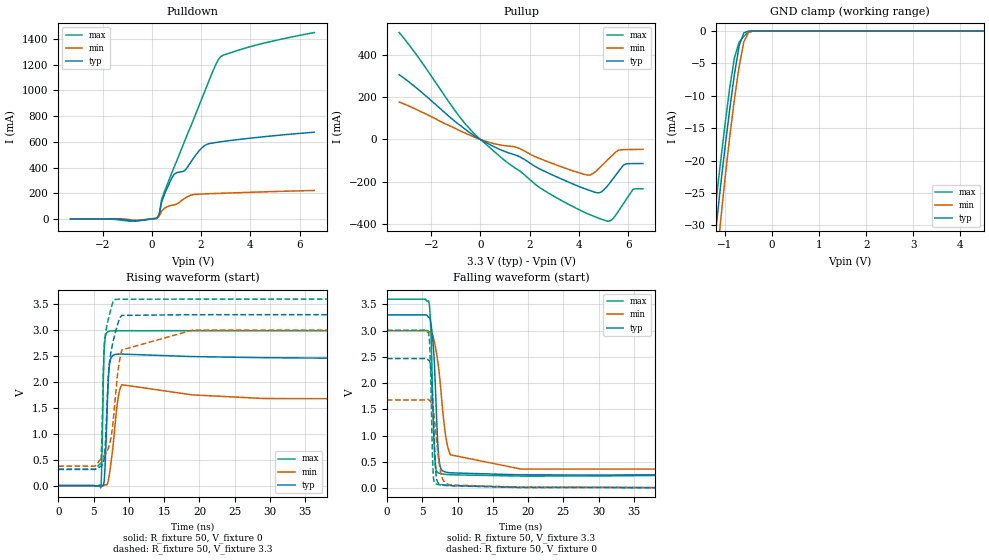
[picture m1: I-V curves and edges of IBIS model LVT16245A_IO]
|   TEXAS INSTRUMENTS INCORPORATED
|   Advanced Bus Interface Group
|   IBIS Model of SN74LVT16245A
|   3.3-V ABT 16-BIT TRANSCEIVER WITH 3-STATE OUTPUTS
[IBIS Ver]   2.1
[File Name]   sn74lvt16245a.ibs
[File Rev]   1.0
[Date]   05/30/2000
[Source]   File originated at Texas Instruments, Inc.
[Notes]   The following is an IBIS list for the LVT16245A.
|   - All test data contained in this file are derived from
|   hspice(tm) simulations.
|   -  This file may be incomplete or may not be fully compliant
   with the IBIS specification. It will be replaced with a
   version that is IBIS Revision 3.2 compliant and is complete
   and accurate. Please email all questions and comments to
   sllibis@ti.com.
[Disclaimer] Property of Texas Instruments Incorporated.  Unauthorized
   reproduction and/or distribution is strictly prohibited.
   This product is protected under copyright law.
   Created 1996, (C) Copyright 1996, Texas Instruments Inc.,
   All Rights Reserved
   UNLESS THERE IS A SIGNED, WRITTEN AGREEMENT TO THE
   CONTRARY, TEXAS INSTRUMENTS ("TI") IS PROVIDING THE IBIS
   MODELS "AS IS" AND WITHOUT ANY WARRANTY, EXPRESSED OR
   IMPLIED.  TI assumes no liability for:
   1) the accuracy of the IBIS models provided to your
   company;
   2) the proper functioning of these IBIS models in your
   design or for any resulting applications; or
   3) infringement of patents, copyrights or intellectual
   property rights resulting from your use of these IBIS
   models.
   TI provides IBIS Models as a service to our customers.
   You and your company shall not distribute, sell or give
   these models to anyone else without prior written
   permission from TI.
   TI reserves the right to make changes to our products or
   to discontinue any semiconductor product or service
   without notice, and advises our customers to obtain the
   latest version of relevant information to verify, before
   placing orders, that the information being relied on is
   current.
   Please be aware that your receipt and use of the IBIS
   information provided shall serve as acceptance of these
   terms and conditions.  If you do not accept these terms,
   you should return or destroy the IBIS models and any
   other accompanying information immediately.
[Component]   LVT16245A_DL
[manufacturer]   Texas Instruments, Inc.
[Package]
|   typ   min   max
R_pkg   0.048   0.038   0.053
L_pkg   6.046nH   5.084nH   7.968nH
C_pkg   0.813pF   0.569pF   1.157pF
[Pin] signal_name   model_name   R_pin   L_pin   C_pin
1   1DIR   NC   0.046   7.968nH   1.017pF
2   1B1   LVT16245A_IO  0.044   7.299nH   1.157pF
3   1B2   LVT16245A_IO  0.043   6.765nH   1.058pF
4   GND   GND   0.041   6.269nH   0.933pF
5   1B3   LVT16245A_IO  0.038   5.856nH   0.829pF
6   1B4   LVT16245A_IO  0.046   5.802nH   0.79pF
7   VCC   POWER   0.05   5.656nH   0.738pF
8   1B5   LVT16245A_IO  0.053   5.5nH   0.643pF
9   1B6   LVT16245A_IO  0.052   5.304nH   0.606pF
10   GND   GND   0.053   5.189nH   0.583pF
11   1B7   LVT16245A_IO  0.051   5.084nH   0.569pF
12   1B8   LVT16245A_IO  0.053   5.862nH   0.833pF
13   2B1   LVT16245A_IO  0.053   5.862nH   0.833pF
14   2B2   LVT16245A_IO  0.051   5.084nH   0.569pF
15   GND   GND   0.053   5.189nH   0.583pF
16   2B3   LVT16245A_IO  0.052   5.304nH   0.606pF
17   2B4   LVT16245A_IO  0.053   5.5nH   0.643pF
18   VCC   POWER   0.05   5.656nH   0.738pF
19   2B5   LVT16245A_IO  0.046   5.802nH   0.79pF
20   2B6   LVT16245A_IO  0.038   5.856nH   0.829pF
21   GND   GND   0.041   6.269nH   0.933pF
22   2B7   LVT16245A_IO  0.043   6.765nH   1.058pF
23   2B8   LVT16245A_IO  0.044   7.299nH   1.157pF
24   2DIR   NC   0.046   7.968nH   1.017pF
25   2NOE   NC   0.046   7.968nH   1.017pF
26   2A8   LVT16245A_IO  0.044   7.299nH   1.157pF
27   2A7   LVT16245A_IO  0.043   6.765nH   1.058pF
28   GND   GND   0.041   6.269nH   0.933pF
29   2A6   LVT16245A_IO  0.038   5.856nH   0.829pF
30   2A5   LVT16245A_IO  0.046   5.802nH   0.79pF
31   VCC   POWER   0.05   5.656nH   0.738pF
32   2A4   LVT16245A_IO  0.053   5.5nH   0.643pF
33   2A3   LVT16245A_IO  0.052   5.304nH   0.606pF
34   GND   LVT16245A_IO  0.053   5.189nH   0.583pF
35   2A2   LVT16245A_IO  0.051   5.084nH   0.569pF
36   2A1   LVT16245A_IO  0.053   5.862nH   0.833pF
37   1A8   LVT16245A_IO  0.053   5.862nH   0.833pF
38   1A7   LVT16245A_IO  0.051   5.084nH   0.569pF
39   GND   GND   0.053   5.189nH   0.583pF
40   1A6   LVT16245A_IO  0.052   5.304nH   0.606pF
41   1A5   LVT16245A_IO  0.053   5.5nH   0.643pF
42   VCC   POWER   0.05   5.656nH   0.738pF
43   1A4   LVT16245A_IO  0.046   5.802nH   0.79pF
44   1A3   LVT16245A_IO  0.038   5.856nH   0.829pF
45   GND   GND   0.041   6.269nH   0.933pF
46   1A2   LVT16245A_IO  0.043   6.765nH   1.058pF
47   1A1   LVT16245A_IO  0.044   7.299nH   1.157pF
48   1NOE   NC   0.046   7.967nH   1.017pF
[Component]   LVT16245A_DGG
[manufacturer]   Texas Instruments, Inc.
[Package]
|   typ   min   max
R_pkg   0.044   0.038   0.051
L_pkg   3.019nH   2.486nH   4.099nH
C_pkg   0.507pF   0.334pF   0.809pF
[Pin]   signal_name   model_name   R_pin   L_pin   C_pin
1   1DIR   NC   0.041   4.017nH   0.759pF
2   1B1   LVT16245A_IO   0.042   3.737nH   0.792pF
3   1B2   LVT16245A_IO   0.042   3.48nH   0.661pF
4   GND   GND   0.038   3.131nH   0.575pF
5   1B3   LVT16245A_IO   0.047   3.122nH   0.566pF
6   1B4   LVT16245A_IO   0.043   2.948nH   0.504pF
7   VCC   POWER   0.045   2.845nH   0.397pF
8   1B5   LVT16245A_IO   0.049   2.835nH   0.394pF
9   1B6   LVT16245A_IO   0.048   2.715nH   0.378pF
10   GND   GND   0.05   2.664nH   0.363pF
11   1B7   LVT16245A_IO   0.05   2.585nH   0.348pF
12   1B8   LVT16245A_IO   0.049   2.55nH   0.337pF
13   2B1   LVT16245A_IO   0.049   2.541nH   0.336pF
14   2B2   LVT16245A_IO   0.05   2.574nH   0.348pF
15   GND   GND   0.049   2.618nH   0.359pF
16   2B3   LVT16245A_IO   0.046   2.671nH   0.375pF
17   2B4   LVT16245A_IO   0.045   2.754nH   0.389pF
18   VCC   POWER   0.044   2.823nH   0.45pF
19   2B5   LVT16245A_IO   0.042   2.968nH   0.503pF
20   2B6   LVT16245A_IO   0.051   3.108nH   0.535pF
21   GND   GND   0.042   3.175nH   0.587pF
22   2B7   LVT16245A_IO   0.041   3.449nH   0.678pF
23   2B8   LVT16245A_IO   0.044   3.766nH   0.804pF
24   2DIR   NC   0.043   4.065nH   0.761pF
25   2NOE   NC   0.041   3.994nH   0.757pF
26   2A8   LVT16245A_IO   0.039   3.649nH   0.789pF
27   2A7   LVT16245A_IO   0.038   3.362nH   0.66pF
28   GND   GND   0.038   3.082nH   0.574pF
29   2A6   LVT16245A_IO   0.044   2.99nH   0.522pF
30   2A5   LVT16245A_IO   0.041   2.917nH   0.495pF
31   VCC   POWER   0.043   2.82nH   0.448pF
32   2A4   LVT16245A_IO   0.043   2.699nH   0.385pF
33   2A3   LVT16245A_IO   0.045   2.628nH   0.372pF
34   GND   LVT16245A_IO   0.046   2.556nH   0.356pF
35   2A2   LVT16245A_IO   0.046   2.495nH   0.344pF
36   2A1   LVT16245A_IO   0.047   2.487nH   0.334pF
37   1A8   LVT16245A_IO   0.047   2.49nH   0.335pF
38   1A7   LVT16245A_IO   0.046   2.486nH   0.343pF
39   GND   GND   0.045   2.566nH   0.356pF
40   1A6   LVT16245A_IO   0.044   2.639nH   0.374pF
41   1A5   LVT16245A_IO   0.043   2.701nH   0.386pF
42   VCC   POWER   0.043   2.817nH   0.45pF
43   1A4   LVT16245A_IO   0.041   2.935nH   0.501pF
44   1A3   LVT16245A_IO   0.047   3.035nH   0.529pF
45   GND   GND   0.043   3.171nH   0.589pF
46   1A2   LVT16245A_IO   0.04   3.415nH   0.682pF
47   1A1   LVT16245A_IO   0.043   3.741nH   0.809pF
48   1NOE   NC   0.044   4.099nH   0.764pF
| Models and submodels in the file (1): LVT16245A_IO (I/O)
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|   Model LVT16245A_IO
[Model]   LVT16245A_IO
|Signals
Model_type  I/O
Polarity   Non-Inverting
Enable   Active-Low
Vinl = 0.8V
Vinh = 2.0V
Vmeas= 1.5V
Cref = 50pf
Rref = 500
Vref = 0V
| variable   typ   min   max
C_comp   11p   NA   NA
[Temperature Range]   50   100   0
[Voltage range]   3.3   3   3.6
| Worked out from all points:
|   slope of the pulldown table from 0 to 0.495 V, typ, clamps not added: 2.73 ohm
|   slope of the pullup table from 0 to 0.495 V, typ, clamps not added: 16 ohm
|   GND clamp passes 1 mA (typ) near -0.63 V on its own axis
|   rising waveform, R_fixture 50, V_fixture 0: 20-80 % time 395ps typ, 805ps min, 252ps max; typ from 0.003 V to 2.45 V
|   falling waveform, R_fixture 50, V_fixture 3.3: 20-80 % time 613ps typ, 1.31ns min, 403ps max; typ from 3.3 V to 0.317 V
|   rising waveform, R_fixture 50, V_fixture 3.3: 20-80 % time 938ps typ, 1.34ns min, 515ps max; typ from 0.318 V to 3.3 V
|   falling waveform, R_fixture 50, V_fixture 0: 20-80 % time 471ps typ, 847ps min, 306ps max; typ from 2.47 V to 0.004 V
|Process range|   weak   strong
[Pullup]
|   50C:3.3V:   100C:3V:weak   0C:3.6V:strong
|   Voltage   I(typ)   I(min)   I(max)
-3.3V     306.3mA    177.3mA    505.4mA
-600mV    46.76mA    29.06mA    71.37mA
500mV     -31.2mA    -18.07mA   -50.75mA
1.5V      -76.63mA   -38.87mA   -141.3mA
2.5V      -144.5mA   -94.5mA    -234.5mA
4.4V      -239.6mA   -168.7mA   -353.5mA
4.8V      -252.4mA   -138.7mA   -372mA
5.2V      -213.8mA   -92.38mA   -386.9mA
5.4V      -183.6mA   -69.91mA   -372.1mA
5.8V      -122.4mA   -48.4mA    -305.3mA
6.2V      -114mA     -47.28mA   -235.6mA
6.6V      -113.7mA   -46.83mA   -232.9mA
[Pulldown]
|   50C:3.3V:   100C:3V:weak   0C:3.6V:strong
|   Voltage   I(typ)   I(min)   I(max)
-3.3V     -454.1uA   -370.1uA   -647.8uA
-800mV    -13.94mA   -8.128mA   -18.68mA
200mV     4.653mA    3.739mA    5.357mA
300mV     33.76mA    20.7mA     29.52mA
400mV     132.5mA    59.25mA    151.5mA
900mV     345.3mA    108.8mA    399.2mA
1.4V      389.3mA    167.7mA    636.1mA
2.1V      563.8mA    194.3mA    969.5mA
2.6V      594.8mA    197.9mA    1.202A
2.8V      600.7mA    199.3mA    1.263A
4.3V      634.6mA    209mA      1.357A
6.6V      675mA      221.3mA    1.451A
[GND Clamp]
|   50C:3.3V:   100C:3V:weak   0C:3.6V:strong
|   Voltage   I(typ)   I(min)   I(max)
-3.3V     -468.6mA   -461.1mA   -471.3mA
-1.3V     -38.64mA   -46.31mA   -33.42mA
-1.2V     -31.14mA   -37.51mA   -26.9mA
-1.1V     -24.32mA   -29.83mA   -20.58mA
-1V       -18.02mA   -22.8mA    -14.47mA
-900mV    -12.13mA   -16.38mA   -8.783mA
-800mV    -6.727mA   -10.6mA    -4.173mA
-700mV    -2.315mA   -5.519mA   -1.718mA
-600mV    -302.6uA   -1.698mA   -835uA
-500mV    -9.036uA   -201.5uA   -187uA
-400mV    -337.9nA   -15.14uA   -80.99nA
6.6V      407.7nA    13.2uA     3.725nA
[ramp]
| variable   typ   min   max
dV/dt_r   1.5296E+00/4.1490E-10  1.2079E+00/9.6417E-10  1.8192E+00/2.5208E-10
dV/dt_f   1.8129E+00/6.1737E-10  1.5085E+00/1.2204E-09  2.0123E+00/4.1438E-10
[Rising Waveform]
R_fixture = 50
V_fixture = 0
V_fixture_min = 0
V_fixture_max = 0
L_fixture= 0nH
C_fixture= 0pF
|   50C:3.3V:   100C:3V:weak   0C:3.6V:strong
|   Time   V(typ)   V(min)   V(max)
0s        3.287mV    2.224mV    5.201mV
6ns       16.07mV    4.52mV     -40.33mV
6.15ns    6.625mV    9.386mV    377.8mV
6.4ns     9.771mV    12.93mV    2.189V
6.5ns     93.11mV    16.17mV    2.626V
7.15ns    2.199V     150.6mV    2.979V
8.4ns     2.54V      1.626V     2.99V
9ns       2.54V      1.949V     2.99V
29ns      2.47V      1.683V     2.991V
100ns     2.451V     1.68V      2.991V
[Falling Waveform]
R_fixture = 50
V_fixture = 3.3
V_fixture_min = 3
V_fixture_max = 3.6
L_fixture= 0nH
C_fixture= 0pF
|   50C:3.3V:   100C:3V:weak   0C:3.6V:strong
|   Time   V(typ)   V(min)   V(max)
0s        3.3V       3V         3.6V
5.9ns     3.255V     2.992V     3.566V
6.25ns    3.127V     2.951V     2.905V
6.8ns     2.144V     2.733V     549mV
7.2ns     860.9mV    2.408V     293.8mV
7.55ns    406.9mV    1.995V     276.1mV
8.3ns     305.2mV    1.008V     260.4mV
9ns       289.2mV    632.2mV    252.6mV
19ns      250.9mV    361.8mV    227.4mV
100ns     317.2mV    372.7mV    316.4mV
[Rising Waveform]
R_fixture = 50
V_fixture = 3.3
V_fixture_min = 3
V_fixture_max = 3.6
L_fixture= 0nH
C_fixture= 0pF
|   50C:3.3V:   100C:3V:weak   0C:3.6V:strong
|   Time   V(typ)   V(min)   V(max)
0s        317.5mV    378.5mV    316.1mV
6ns       374.8mV    515.6mV    427.5mV
6.15ns    388.6mV    540.4mV    821.6mV
6.4ns     461.9mV    572.9mV    2.31V
6.55ns    592.5mV    594.3mV    2.777V
7.15ns    2.235V     753.7mV    3.25V
7.95ns    2.89V      1.507V     3.591V
9ns       3.287V     2.62V      3.598V
19ns      3.3V       3.001V     3.6V
100ns     3.3V       3V         3.6V
[Falling Waveform]
R_fixture = 50
V_fixture = 0
V_fixture_min = 0
V_fixture_max = 0
L_fixture= 0nH
C_fixture= 0pF
|   50C:3.3V:   100C:3V:weak   0C:3.6V:strong
|   Time   V(typ)   V(min)   V(max)
0s        2.468V     1.678V     3.009V
5.9ns     2.434V     1.687V     2.956V
6.15ns    2.358V     1.652V     2.415V
6.4ns     1.907V     1.606V     894.7mV
6.55ns    1.439V     1.516V     281.6mV
6.9ns     358.4mV    1.09V      80.15mV
7.1ns     139.2mV    816.1mV    69.56mV
7.8ns     62.79mV    199mV      56.51mV
9ns       46.43mV    57.06mV    43.13mV
100ns     3.552mV    2.862mV    5.313mV
